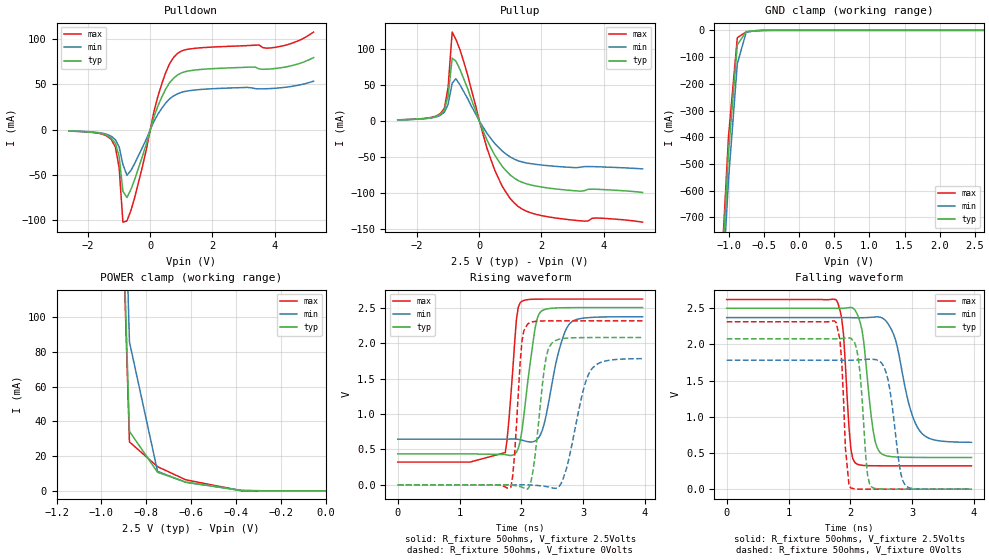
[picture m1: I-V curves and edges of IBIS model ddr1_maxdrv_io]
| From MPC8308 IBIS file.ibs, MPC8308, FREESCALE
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[Model]   ddr1_maxdrv_io   |
Model_type   I/O
Vinl = 1.22
Vinh = 1.28
Vmeas = 1.25
Cref = 1E-11
Rref = 50
Vref = 1.25
| variable   typ   min   max
C_comp   1.17p   1.10p   1.23p
[Model Spec]
| subparameter   typ   min   max
S_overshoot_high  3.300   3.135   3.465
S_overshoot_low   -200.00m  -100.00m  -300.00m
D_overshoot_high  4.000   4.000   4.000
D_overshoot_low   -1.000   -1.000   -1.000
D_overshoot_time  1.000n   1.000n   1.000n
| variable   typ   min   max
[Temperature Range]   25.0   -40.0   125.0
| variable   typ   min   max
[Pullup Reference]   2.500V   2.375V   2.625V
| variable   typ   min   max
[Pulldown Reference]   0.000V   0.000V   0.000V
| variable   typ   min   max
[POWER_Clamp_Reference]   2.500V   2.375V   2.625V
| variable   typ   min   max
[GND_Clamp_Reference]   0.000V   0.000V   0.000V
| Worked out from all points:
|   slope of the pulldown table from 0 to 0.375 V, typ, clamps not added: 10.3 ohm
|   slope of the pullup table from 0 to 0.375 V, typ, clamps not added: 10.1 ohm
|   GND clamp passes 1 mA (typ) near -0.59 V on its own axis
|   POWER clamp passes 1 mA (typ) near -0.42 V on its own axis
|   rising waveform, R_fixture 50ohms, V_fixture 2.5Volts: 20-80 % time 179ps typ, 250ps min, 121ps max; typ from 0.438 V to 2.5 V
|   rising waveform, R_fixture 50ohms, V_fixture 0Volts: 20-80 % time 153ps typ, 264ps min, 99.6ps max; typ from 0 V to 2.08 V
|   falling waveform, R_fixture 50ohms, V_fixture 2.5Volts: 20-80 % time 154ps typ, 272ps min, 98.4ps max; typ from 2.5 V to 0.438 V
|   falling waveform, R_fixture 50ohms, V_fixture 0Volts: 20-80 % time 104ps typ, 160ps min, 79.7ps max; typ from 2.08 V to 0 V
[Pulldown]
| pulldown in the table = pulldown subtract gnd_clamp
|Voltage   I(typ)   I(min)   I(max)
-2.62V    -1.502mA   -1.359mA   -1.575mA
-1.25V    -9.33mA    -7.387mA   -10.97mA
-1.12V    -15.17mA   -11.09mA   -19.3mA
-1V       -29.77mA   -19.18mA   -42.3mA
-880mV    -68.05mA   -38.43mA   -102.2mA
-750mV    -75mA      -50.49mA   -100.8mA
-250mV    -29.21mA   -19.48mA   -40.4mA
250mV     26.55mA    17.35mA    37.4mA
620mV     51.84mA    33.98mA    72.8mA
880mV     60.51mA    39.67mA    84.41mA
4V        67.52mA    45.74mA    90.9mA
5.25V     79.58mA    53.57mA    107.8mA
[Pullup]
| pullup in the table = pullup subtract power_clamp
|Voltage   I(typ)   I(min)   I(max)
-2.62V    1.701mA    1.624mA    1.779mA
-1.5V     5.184mA    4.685mA    5.604mA
-1.12V    15.32mA    12.25mA    17.83mA
-1V       35.28mA    23.42mA    47.06mA
-870mV    87.71mA    52.83mA    124mA
-750mV    83.62mA    59.03mA    114mA
-370mV    44.94mA    31.14mA    63.86mA
380mV     -37.7mA    -24.58mA   -54.22mA
750mV     -63.71mA   -42.16mA   -91.59mA
1.13V     -79.59mA   -53.09mA   -114.3mA
2.38V     -94.19mA   -62.81mA   -134.6mA
5.25V     -99.46mA   -66.66mA   -140.9mA
[GND_clamp]
|Voltage   I(typ)   I(min)   I(max)
-2.625V   -9.497A    -9.494A    -9.517A
-1.125V   -1.057A    -1.145A    -1.012A
-1V       -454.7mA   -557.3mA   -396.5mA
-875mV    -54.6mA    -124.7mA   -27.53mA
-750mV    -4.635mA   -8.012mA   -5.794mA
-625mV    -1.367mA   -1.259mA   -1.854mA
-500mV    -191.1uA   -225.6uA   -219.2uA
2.625V    45.37nA    27.37uA    16.83pA
[POWER_clamp]
|Voltage   I(typ)   I(min)   I(max)
-2.375V   9.526A     9.538A     9.599A
-1.125V   1.078A     1.196A     1.069A
-875mV    34.28mA    85.75mA    28.2mA
-750mV    10.75mA    11.29mA    13.96mA
-625mV    5.151mA    4.938mA    6.448mA
-375mV    135.8uA    350uA      84.92uA
0V        255.3pA    14.06nA    16.83pA
[Ramp]
|Voltage   I(typ)   I(min)   I(max)
dV/dt_f   1.24/153.438p 1.04/272.746p 1.39/97.185p
dV/dt_r   1.28/157.817p 1.10/272.818p 1.43/100.724p
R_load=50ohms
| R_load was connected to ground for Ramp_up test and power for Ramp_dn test
[Rising_Waveform]
R_fixture=50ohms
V_fixture=2.5Volts
V_fixture_min=2.375Volts
V_fixture_max=2.625Volts
|C_fixture=1E-15f
|L_fixture=1E-15h
|C_dut=1E-15fh
|R_dut=0.001ohm
|L_dut=1E-12h
|time   V(typ)   V(min)   V(max)
0s        438.3mV    645.3mV    322.7mV
1.74ns    428.8mV    645.5mV    456.1mV
1.8ns     417.2mV    646.4mV    930.9mV
1.92ns    460.9mV    645.7mV    2.337V
2.01ns    770.5mV    630.7mV    2.59V
2.22ns    2.202V     619mV      2.619V
2.31ns    2.439V     710.6mV    2.62V
2.61ns    2.497V     1.901V     2.62V
2.79ns    2.499V     2.281V     2.621V
3.96ns    2.5V       2.371V     2.621V
[Rising_Waveform]
R_fixture=50ohms
V_fixture=0Volts
|C_fixture=1E-15f
|L_fixture=1E-15h
|C_dut=1E-15fh
|R_dut=0.001ohm
|L_dut=1E-12h
|time   V(typ)   V(min)   V(max)
0s        6.447nV    581nV      144.8pV
1.83ns    -1.746mV   5.208uV    -32.2mV
1.89ns    -8.06mV    918.6uV    425.9mV
2.01ns    -31.4mV    2.261mV    2.03V
2.1ns     -59.48mV   1.369mV    2.268V
2.19ns    209.8mV    -2.815mV   2.301V
2.4ns     1.798V     -21.92mV   2.312V
2.58ns    2.046V     -42.64mV   2.313V
3.12ns    2.078V     1.613V     2.313V
3.96ns    2.078V     1.781V     2.313V
[Falling_Waveform]
R_fixture=50ohms
V_fixture=2.5Volts
V_fixture_min=2.375Volts
V_fixture_max=2.625Volts
|C_fixture=1E-15f
|L_fixture=1E-15h
|C_dut=1E-15fh
|R_dut=0.001ohm
|L_dut=1E-12h
|time   V(typ)   V(min)   V(max)
0s        2.5V       2.371V     2.621V
1.77ns    2.498V     2.371V     2.619V
1.86ns    2.498V     2.371V     2.362V
1.98ns    2.509V     2.371V     830.8mV
2.07ns    2.481V     2.369V     372mV
2.19ns    2.194V     2.369V     330.1mV
2.4ns     667.1mV    2.38V      323.3mV
2.52ns    481.4mV    2.364V     322.8mV
3.12ns    438.6mV    809mV      322.7mV
3.96ns    438.3mV    647.2mV    322.7mV
[Falling_Waveform]
R_fixture=50ohms
V_fixture=0Volts
|C_fixture=1E-15f
|L_fixture=1E-15h
|C_dut=1E-15fh
|R_dut=0.001ohm
|L_dut=1E-12h
|time   V(typ)   V(min)   V(max)
0s        2.078V     1.782V     2.313V
1.77ns    2.077V     1.782V     2.303V
1.83ns    2.08V      1.782V     2.074V
2.01ns    2.086V     1.782V     16.06mV
2.13ns    1.805V     1.786V     1.284mV
2.28ns    187.6mV    1.795V     191.8uV
2.34ns    33.69mV    1.795V     91.03uV
2.58ns    957.4uV    1.608V     4.753uV
2.88ns    80.61uV    66.32mV    102.5nV
3.96ns    10.98nV    30.58uV    -7.376nV
